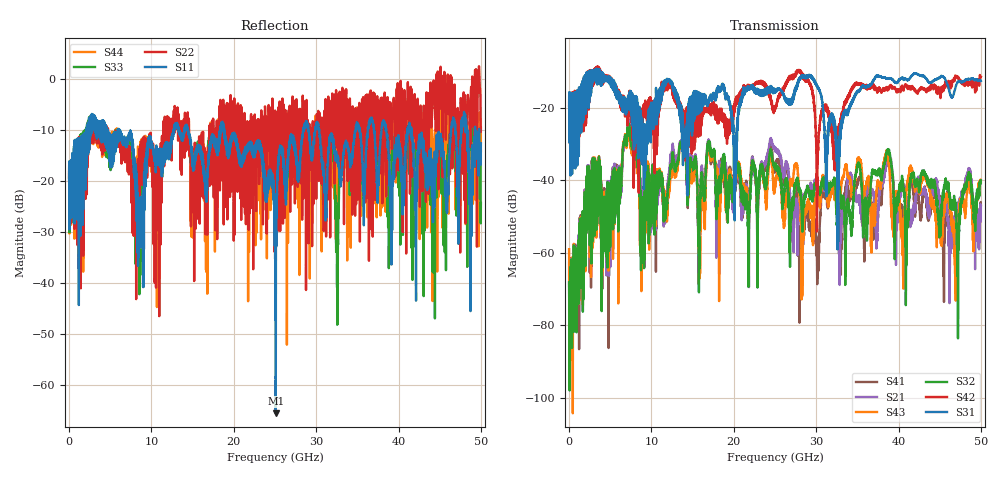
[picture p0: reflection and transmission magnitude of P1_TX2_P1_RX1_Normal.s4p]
!Keysight Technologies,N5225B,MY57041031,A.13.20.10
!Date: Friday, May 31, 2019 11:13:48
!Correction: S11(Full 4 Port(1,2,3,4))
!S12(Full 4 Port(1,2,3,4))
!S13(Full 4 Port(1,2,3,4))
!S14(Full 4 Port(1,2,3,4))
!S21(Full 4 Port(1,2,3,4))
!S22(Full 4 Port(1,2,3,4))
!S23(Full 4 Port(1,2,3,4))
!S24(Full 4 Port(1,2,3,4))
!S31(Full 4 Port(1,2,3,4))
!S32(Full 4 Port(1,2,3,4))
!S33(Full 4 Port(1,2,3,4))
!S34(Full 4 Port(1,2,3,4))
!S41(Full 4 Port(1,2,3,4))
!S42(Full 4 Port(1,2,3,4))
!S43(Full 4 Port(1,2,3,4))
!S44(Full 4 Port(1,2,3,4))
!S4P File: Measurements: <S11,S12,S13,S14>,
!<S21,S22,S23,S24>,
!<S31,S32,S33,S34>,
!<S41,S42,S43,S44>:
# Hz S  dB  R 50.0
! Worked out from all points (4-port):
!   5000 points, 10 MHz to 50 GHz, reference 50 ohm
!   strongest paths, dB at 10 MHz, 12.51 GHz, 25.01 GHz, 37.51 GHz, 50 GHz:
!     S31: -19.5, -13.0, -15.4, -11.1, -12.5
!     S42: -19.5, -14.7, -20.1, -15.1, -11.4
!     S32: -68.2, -34.5, -36.2, -38.2, -40.1
!     S43: -59.0, -37.0, -40.9, -40.8, -40.6
!     S21: -62.8, -32.0, -31.5, -49.3, -47.1
!     S41: -68.1, -34.2, -36.6, -42.3, -46.8
!   lowest |S11| = -65.4 dB at 25.1 GHz (marker M1), VSWR 1.00, Z = 50 + j0.0346 ohm
!   |S11| at or under -10 dB: 6.091 GHz to 12.71 GHz (6.616 GHz wide, 70.4 % of centre); 18.82 GHz to 28.43 GHz (9.605 GHz wide, 40.7 % of centre); 41.58 GHz to 46.39 GHz (4.81 GHz wide, 10.9 % of centre)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
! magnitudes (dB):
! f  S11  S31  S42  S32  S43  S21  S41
! 10 MHz  -19.8  -19.5  -19.5  -68.2  -59.0  -62.8  -68.1
! 7.28 GHz  -11.0  -17.7  -16.4  -24.4  -24.8  -23.4  -23.9
! 8.87 GHz  -26.7  -24.2  -20.3  -45.1  -55.5  -41.9  -51.5
! 13.86 GHz  -11.1  -25.9  -23.7  -27.6  -28.0  -27.0  -27.4
! 25.1 GHz  -65.4  -15.1  -19.8  -35.4  -39.1  -31.0  -34.9
! 28.12 GHz  -15.0  -11.3  -10.2  -43.7  -48.8  -44.2  -53.5
! 50 GHz  -12.6  -12.5  -11.4  -40.1  -40.6  -47.1  -46.8
